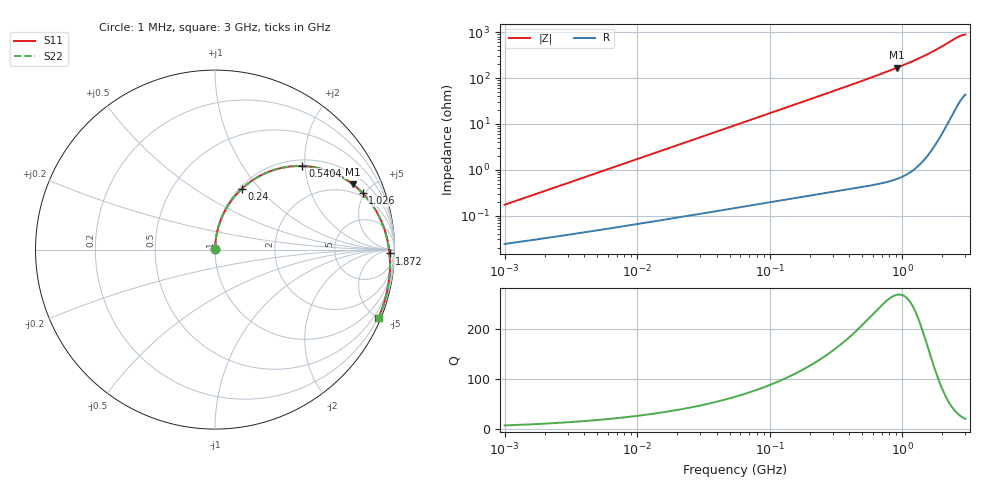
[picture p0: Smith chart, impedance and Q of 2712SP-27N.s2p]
# MHz  S  MA  R  50
!Freq  MagS11  AngS11  MagS21  AngS21  MagS12  AngS12  MagS22  AngS22
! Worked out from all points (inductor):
!   801 points, 1 MHz to 3 GHz, reference 50 ohm
!   read as one part in series: L = 27.1 nH near 1.041 MHz
!   highest Q = 267 at 909.9 MHz (marker M1), where L = 29.3 nH
!   S11 on the Smith chart (normalised r, x): 1 MHz: 1.00, +0.00; 240 MHz: 1.03, +0.80; 540.4 MHz: 1.14, +1.94; 1.026 GHz: 1.72, +4.83; 1.872 GHz: 44, -35; 3 GHz: 0.17, -4.97
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1  0.001662 81.6  0.9998 -0.1  0.9998 -0.1  0.001662 81.6
3.829105  0.006311 85.8  0.9996 -0.4  0.9996 -0.4  0.006311 85.8
14.51587  0.02387 86.7  0.9989 -1.5  0.9989 -1.5  0.02387 86.7
30.16481  0.04953 85.7  0.9977 -3.0  0.9977 -3.0  0.04953 85.7
55.02866  0.09009 83.5  0.9945 -5.5  0.9945 -5.5  0.09007 83.5
82.98494  0.1352 80.9  0.9891 -8.3  0.9891 -8.3  0.1351 80.9
120.2275  0.194 77.4  0.9789 -12.0  0.9789 -12.0  0.1939 77.4
160.7668  0.2558 73.6  0.9644 -15.9  0.9644 -15.9  0.2557 73.6
208.6098  0.3251 69.2  0.9431 -20.4  0.9431 -20.4  0.325 69.2
240.0244  0.3682 66.4  0.927 -23.2  0.927 -23.2  0.3681 66.4
354.783  0.5075 56.8  0.8586 -32.9  0.8586 -32.9  0.5073 56.8
442.2779  0.5944 50.3  0.8011 -39.4  0.8011 -39.4  0.5941 50.3
540.4116  0.6736 43.7  0.736 -46.0  0.736 -46.0  0.6732 43.7
653.7363  0.7451 37.2  0.664 -52.6  0.664 -52.6  0.7446 37.2
790.8254  0.8092 30.4  0.5846 -59.4  0.5846 -59.4  0.8087 30.4
909.9158  0.8504 25.3  0.5233 -64.5  0.5233 -64.5  0.8498 25.3
1026.169  0.8811 20.9  0.4701 -68.8  0.4701 -68.8  0.8804 20.9
1399.956  0.9404 9.6  0.3358 -80.1  0.3358 -80.1  0.9398 9.6
1872.006  0.9725 -1.3  0.2229 -90.7  0.2229 -90.7  0.9721 -1.3
2241.99  0.9829 -8.6  0.1639 -97.5  0.1639 -97.5  0.9829 -8.6
2658.329  0.9871 -16.3  0.1219 -104.3  0.1219 -104.3  0.9878 -16.3
3000  0.9869 -22.7  0.1064 -109.8  0.1064 -109.8  0.9884 -22.7
